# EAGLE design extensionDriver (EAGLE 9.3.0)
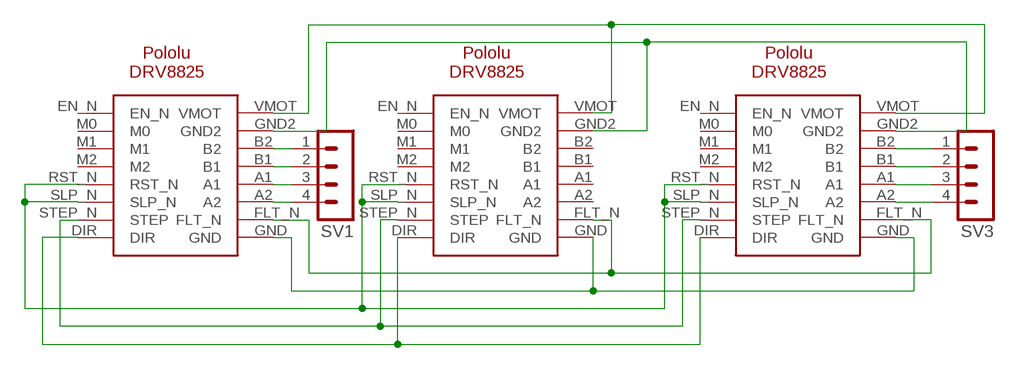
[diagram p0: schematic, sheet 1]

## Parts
SV1  CON-LSTB_MA04-1  [CON-LSTB_MA04-1]
SV3  CON-LSTB_MA04-1  [CON-LSTB_MA04-1]
U$1  POLOLU-DRV8825  [POLOLU-DRV8825]
U$2  POLOLU-DRV8825  [POLOLU-DRV8825]
U$3  POLOLU-DRV8825  [POLOLU-DRV8825]

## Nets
N$1: U$1.VMOT U$2.VMOT U$3.VMOT
N$2: U$1.RST_N U$1.SLP_N U$2.RST_N U$2.SLP_N U$3.RST_N U$3.SLP_N
N$3: U$1.GND2 U$2.GND2 U$3.GND2
N$4: SV3.1 U$3.B2
N$5: U$1.DIR U$2.DIR U$3.DIR
N$6: U$1.STEP_N(STEP) U$2.STEP_N(STEP) U$3.STEP_N(STEP)
N$7: SV1.1 U$1.B2
N$8: U$1.GND U$2.GND U$3.GND
N$9: U$1.FLT_N U$2.FLT_N U$3.FLT_N
N$10: SV1.2 U$1.B1
N$11: SV1.3 U$1.A1
N$12: SV1.4 U$1.A2
N$13: SV3.2 U$3.B1
N$14: SV3.3 U$3.A1
N$15: SV3.4 U$3.A2
Unconnected: U$1.EN_N U$1.M0 U$1.M1 U$1.M2 U$2.A1 U$2.A2 U$2.B1 U$2.B2 U$2.EN_N U$2.M0 U$2.M1 U$2.M2 U$3.EN_N U$3.M0 U$3.M1 U$3.M2

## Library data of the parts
SV1 SV3 = GRBLShieldFabDuino:CON-LSTB_MA04-1: PIN HEADER; OC_FARNELL: unknown; OC_NEWARK: unknown
U$1-U$3 = alvarop-lib:POLOLU-DRV8825

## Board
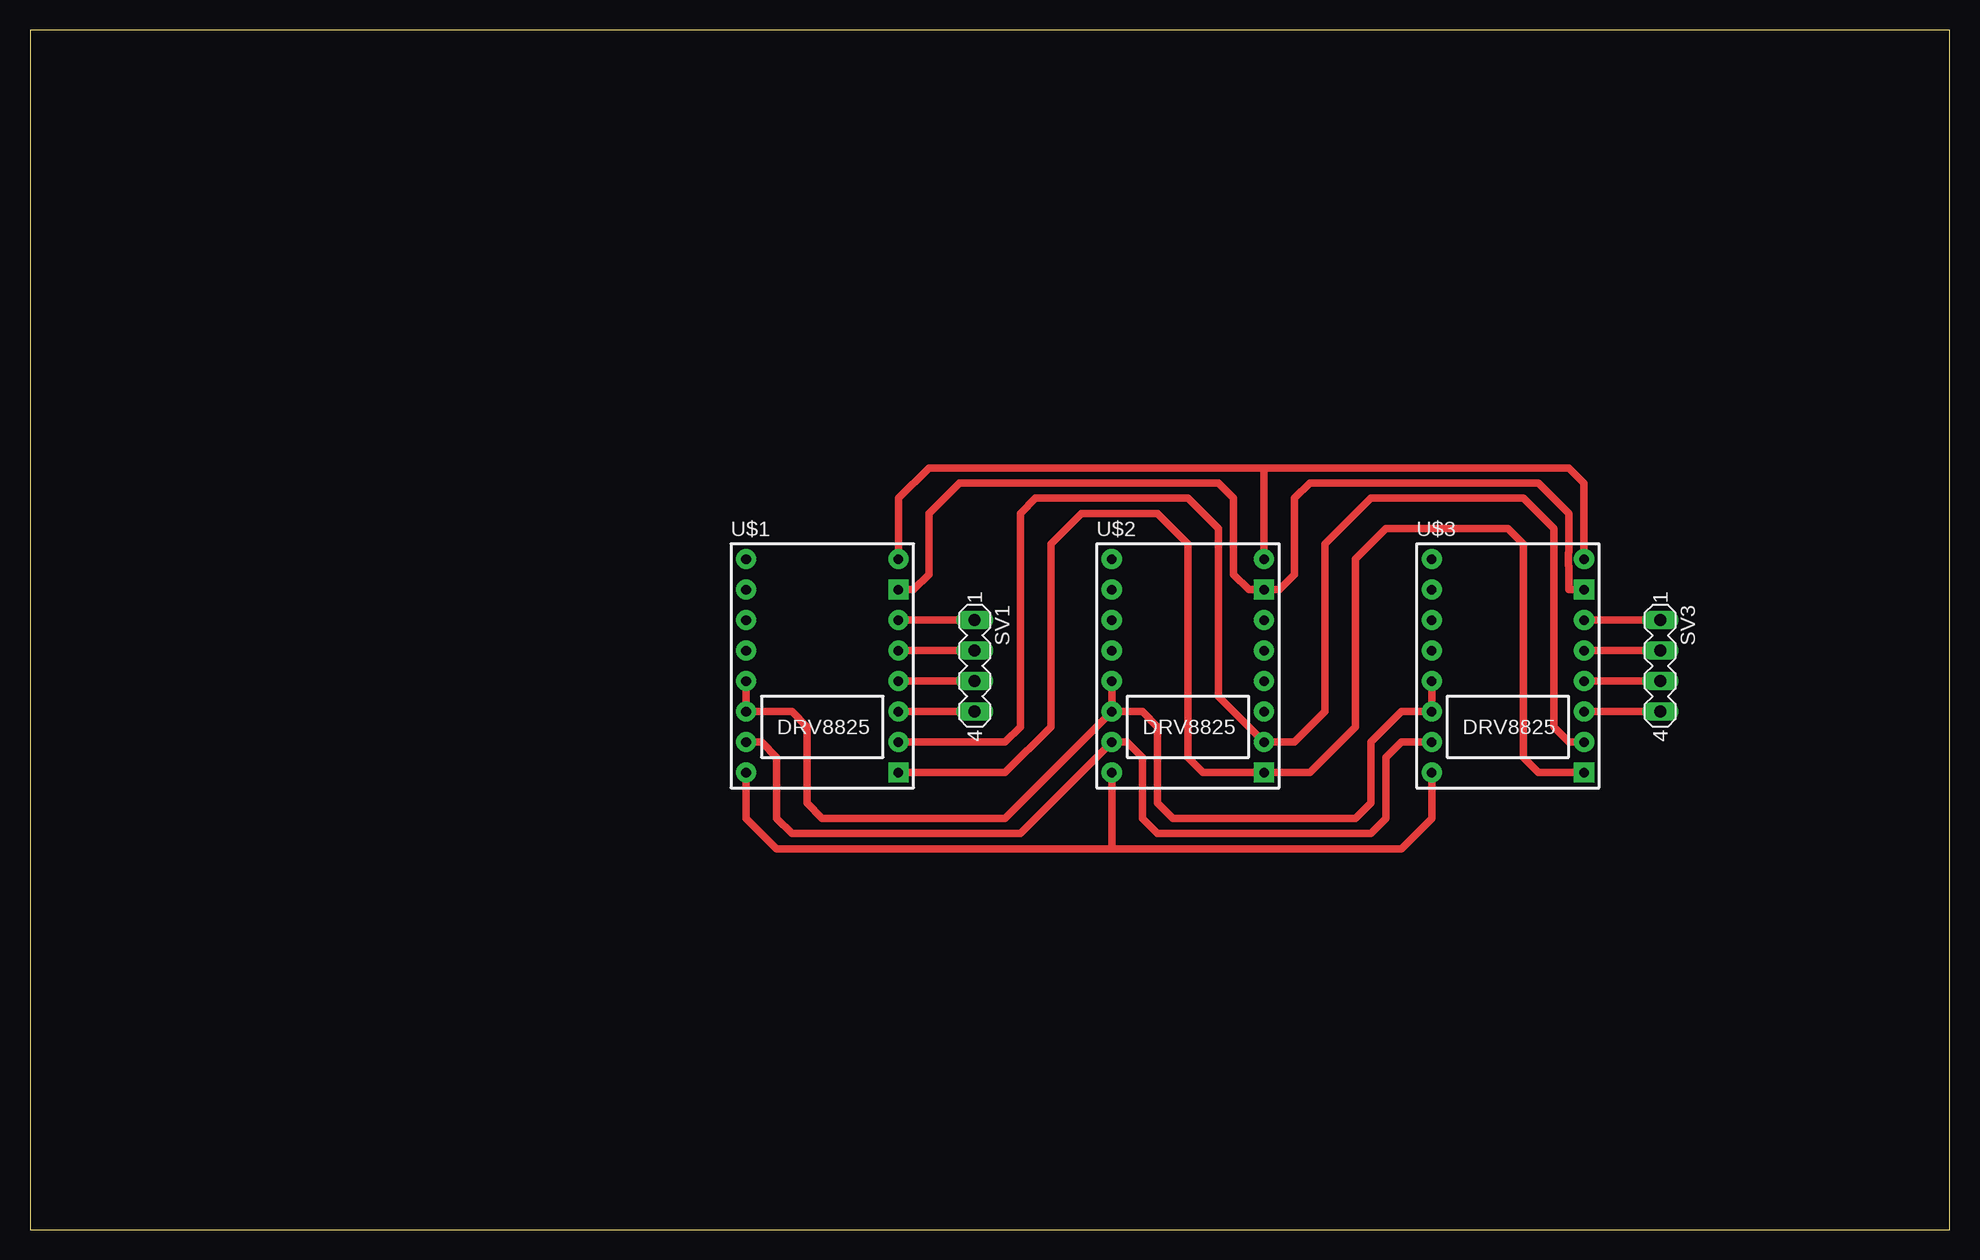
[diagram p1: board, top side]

Size 160 x 100 mm. Coordinates in mm from the lower left corner, seen from the top.
Outline: 0,0 160,0 160,100 0,100 0,0
Copper layers (1*16): Top 0.035mm / dielectric 1.5mm / Bottom 0.035mm
Design rules "default": minimum track width 6mil, minimum drill 0.35mm, track to track 6mil, track to pad 6mil, pad to pad 6mil, via to via 6mil, smd to smd 6mil, copper to edge 40mil, drill to drill 6mil, minimum pad ring 10mil, minimum via ring 8mil, stop-mask expansion 4mil, vias tented up to drill 0mil, thermal gap 10mil

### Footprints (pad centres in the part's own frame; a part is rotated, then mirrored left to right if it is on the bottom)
CON-LSTB_MA04-1 = drill 1.016 long: 1 -3.81,0; 2 -1.27,0; 3 1.27,0; 4 3.81,0
POLOLU-DRV8825 = drill 0.8 pad 1.676: A1 6.35,-1.27; A2 6.35,-3.81; B1 6.35,1.27; B2 6.35,3.81; DIR -6.35,-8.89; EN_N -6.35,8.89; FLT_N 6.35,-6.35; M0 -6.35,6.35; M1 -6.35,3.81; M2 -6.35,1.27; RST_N -6.35,-1.27; SLP_N -6.35,-3.81; STEP_N -6.35,-6.35; VMOT 6.35,8.89 | drill 0.8 pad 1.676 square: GND 6.35,-8.89; GND2 6.35,6.35

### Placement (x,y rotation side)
SV1  78.74,46.99 270 top
SV3  135.89,46.99 270 top
U$1  66.04,46.99 0 top
U$2  96.52,46.99 0 top
U$3  123.19,46.99 0 top

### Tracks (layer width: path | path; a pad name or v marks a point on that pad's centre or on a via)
N$1
  Top 0.61: 102.87,63.5 74.93,63.5 72.39,60.96 U$1.VMOT | 102.87,63.5 128.27,63.5 129.54,62.23 U$3.VMOT | U$2.VMOT 102.87,63.5
N$2
  Top 0.61: U$1.RST_N U$1.SLP_N 63.5,43.18 64.77,41.91 64.77,35.56 66.04,34.29 81.28,34.29 U$2.SLP_N | U$2.RST_N U$2.SLP_N | U$3.RST_N U$3.SLP_N 114.3,43.18 111.76,40.64 111.76,35.56 110.49,34.29 95.25,34.29 93.98,35.56 93.98,41.91 92.71,43.18 U$2.SLP_N
N$3
  Top 0.61: U$1.GND2 73.66,53.34 74.93,54.61 74.93,59.69 77.47,62.23 99.06,62.23 100.33,60.96 100.33,54.61 101.6,53.34 U$2.GND2 104.14,53.34 105.41,54.61 105.41,60.96 106.68,62.23 125.73,62.23 128.27,59.69 128.27,56.44 128.25,56.42 128.25,55.34 128.27,55.32 128.27,53.34 U$3.GND2
N$4
  Top 0.61: SV3.1 U$3.B2
N$5
  Top 0.61: U$1.DIR 59.69,34.29 62.23,31.75 90.17,31.75 | 90.17,31.75 114.3,31.75 116.84,34.29 U$3.DIR | U$2.DIR 90.17,31.75
N$6
  Top 0.61: U$1.STEP_N 60.96,40.64 62.23,39.37 62.23,34.29 63.5,33.02 82.55,33.02 U$2.STEP_N 91.44,40.64 92.71,39.37 92.71,34.29 93.98,33.02 111.76,33.02 113.03,34.29 113.03,39.37 114.3,40.64 U$3.STEP_N
N$7
  Top 0.61: SV1.1 U$1.B2
N$8
  Top 0.61: U$1.GND 81.28,38.1 85.09,41.91 85.09,57.15 87.63,59.69 93.98,59.69 96.52,57.15 96.52,39.37 97.79,38.1 U$2.GND 106.68,38.1 110.49,41.91 110.49,55.88 113.03,58.42 123.19,58.42 124.46,57.15 124.46,39.37 125.73,38.1 U$3.GND
N$9
  Top 0.61: U$1.FLT_N 81.28,40.64 82.55,41.91 82.55,59.69 83.82,60.96 96.52,60.96 99.06,58.42 99.06,44.45 U$2.FLT_N 105.41,40.64 107.95,43.18 107.95,57.15 111.76,60.96 124.46,60.96 127,58.42 127,41.91 128.27,40.64 U$3.FLT_N
N$10
  Top 0.61: SV1.2 U$1.B1
N$11
  Top 0.61: SV1.3 U$1.A1
N$12
  Top 0.61: SV1.4 U$1.A2
N$13
  Top 0.61: SV3.2 U$3.B1
N$14
  Top 0.61: SV3.3 U$3.A1
N$15
  Top 0.61: U$3.A2 SV3.4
